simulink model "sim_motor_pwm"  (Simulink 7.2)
settings: Solver=ode4  SolverMode=SingleTasking  StartTime=0  StopTime=4  FixedStep=2e-5  MaxStep=0.001  RelTol=1e-3  AbsTol=1e-6
InitFcn:
  | initfcn
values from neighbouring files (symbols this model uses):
  b = b_s + b_m*rho*rho    (= 0.0075943)    [initfcn.m]
  f_0_pwm = 50000    [initfcn.m]
  k_t = 0.0172    [initfcn.m]
  k_v = 0.0172    [initfcn.m]
  r_a = 35.2    [initfcn.m]
  rho = 30    [initfcn.m]
  tal_a = l_a/r_a    (= 4.85795454545e-05)    [initfcn.m]
  tal_m = i/b    (= 0.0444425424331)    [initfcn.m]

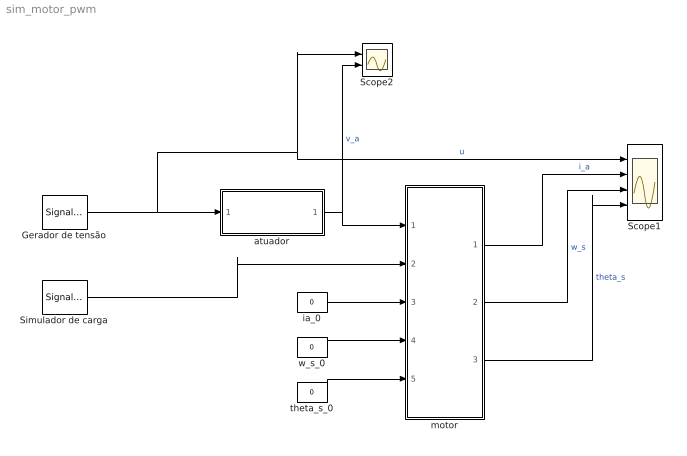
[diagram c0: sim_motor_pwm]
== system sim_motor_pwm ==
  Gerador de tensão : SignalGenerator  WaveForm=square  Amplitude=6  Frequency=0.5
  Scope1 : Scope  NumInputPorts=4
  Scope2 : Scope  NumInputPorts=2
  Simulador de carga : SignalGenerator  WaveForm=square  Amplitude=0.1  Frequency=10
  atuador : Subsystem
  ia_0 : Constant  Value=0  OutDataType=sfix(16)  OutScaling=2^0
  motor : Subsystem
  theta_s_0 : Constant  Value=0  OutDataType=sfix(16)  OutScaling=2^0
  w_s_0 : Constant  Value=0  OutDataType=sfix(16)  OutScaling=2^0
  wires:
  theta_s_0/1 -> motor/5(theta_s_0)
  ia_0/1 -> motor/3(ia_0)
  w_s_0/1 -> motor/4(w_s_0)
  atuador/1(v_a) -> motor/1(v_a), Scope2/2  "v_a"
  Gerador de tensão/1 -> atuador/1(u), Scope1/1, Scope2/1  "u"
  Simulador de carga/1 -> motor/2(tal_l)
  motor/1(i_a) -> Scope1/2  "i_a"
  motor/2(w_s) -> Scope1/3  "w_s"
  motor/3(theta_s) -> Scope1/4  "theta_s"

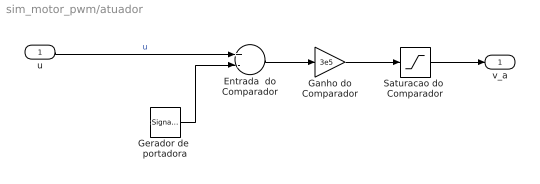
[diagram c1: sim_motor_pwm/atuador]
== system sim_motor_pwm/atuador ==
  u : Inport  OutDataType=sfix(16)  OutScaling=2^0
  Entrada  do Comparador : Sum  Inputs=+-  OutDataType=sfix(16)  OutScaling=2^-10
  Ganho do Comparador : Gain  Gain=3e5  ParameterDataType=sfix(16)  ParameterScaling=2^0  OutDataType=sfix(16)  OutScaling=2^0
  Gerador de  portadora : SignalGenerator  Amplitude=12  Frequency=f_0_pwm
  Saturacao do  Comparador : Saturate  UpperLimit=15  LowerLimit=-15  OutDataType=sfix(16)  OutScaling=2^0
  v_a : Outport  OutDataType=sfix(16)  OutScaling=2^0
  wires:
  Entrada  do Comparador/1 -> Ganho do Comparador/1
  Ganho do Comparador/1 -> Saturacao do  Comparador/1
  Gerador de  portadora/1 -> Entrada  do Comparador/2
  Saturacao do  Comparador/1 -> v_a/1
  u/1 -> Entrada  do Comparador/1  "u"

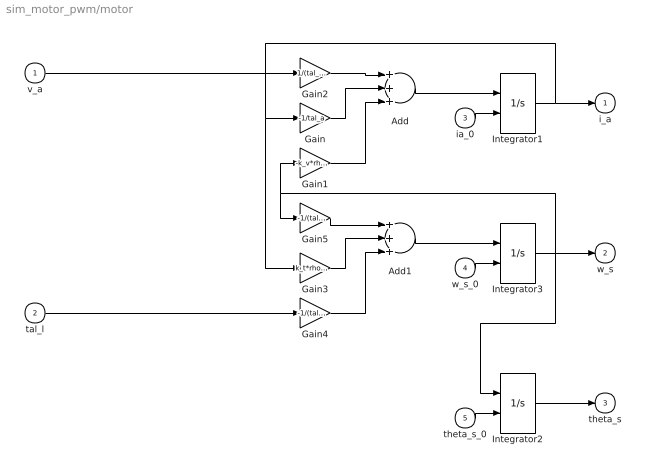
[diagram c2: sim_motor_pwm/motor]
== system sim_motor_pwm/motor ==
  v_a : Inport  OutDataType=sfix(16)  OutScaling=2^0
  tal_l : Inport  Port=2  OutDataType=sfix(16)  OutScaling=2^0
  ia_0 : Inport  Port=3  OutDataType=sfix(16)  OutScaling=2^0
  w_s_0 : Inport  Port=4  OutDataType=sfix(16)  OutScaling=2^0
  theta_s_0 : Inport  Port=5  OutDataType=sfix(16)  OutScaling=2^0
  Add : Sum  Inputs=+++  OutDataType=sfix(16)  OutScaling=2^-10
  Add1 : Sum  Inputs=+++  OutDataType=sfix(16)  OutScaling=2^-10
  Gain : Gain  Gain=-1/tal_a  ParameterDataType=sfix(16)  ParameterScaling=2^0  OutDataType=sfix(16)  OutScaling=2^0
  Gain1 : Gain  Gain=-k_v*rho/(tal_a*r_a)  ParameterDataType=sfix(16)  ParameterScaling=2^0  OutDataType=sfix(16)  OutScaling=2^0
  Gain2 : Gain  Gain=1/(tal_a*r_a)  ParameterDataType=sfix(16)  ParameterScaling=2^0  OutDataType=sfix(16)  OutScaling=2^0
  Gain3 : Gain  Gain=k_t*rho/(tal_m*b)  ParameterDataType=sfix(16)  ParameterScaling=2^0  OutDataType=sfix(16)  OutScaling=2^0
  Gain4 : Gain  Gain=-1/(tal_m*b)  ParameterDataType=sfix(16)  ParameterScaling=2^0  OutDataType=sfix(16)  OutScaling=2^0
  Gain5 : Gain  Gain=-1/(tal_m)  ParameterDataType=sfix(16)  ParameterScaling=2^0  OutDataType=sfix(16)  OutScaling=2^0
  Integrator1 : Integrator  InitialConditionSource=external
  Integrator2 : Integrator  InitialConditionSource=external
  Integrator3 : Integrator  InitialConditionSource=external
  i_a : Outport  OutDataType=sfix(16)  OutScaling=2^0  InitialOutput=0
  w_s : Outport  Port=2  OutDataType=sfix(16)  OutScaling=2^0  InitialOutput=0
  theta_s : Outport  Port=3  OutDataType=sfix(16)  OutScaling=2^0  InitialOutput=0
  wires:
  Integrator1/1 -> i_a/1, Gain/1, Gain3/1
  v_a/1 -> Gain2/1
  Integrator2/1 -> theta_s/1
  ia_0/1 -> Integrator1/2
  theta_s_0/1 -> Integrator2/2
  Gain2/1 -> Add/1
  Gain/1 -> Add/2
  Gain1/1 -> Add/3
  Add/1 -> Integrator1/1
  w_s_0/1 -> Integrator3/2
  Integrator3/1 -> w_s/1, Gain1/1, Gain5/1, Integrator2/1
  Gain5/1 -> Add1/1
  Gain3/1 -> Add1/2
  Gain4/1 -> Add1/3
  Add1/1 -> Integrator3/1
  tal_l/1 -> Gain4/1
